TYPE APCst :
STRUCT
	Enable_b	:	BOOL	;	//	
	P1ZeroOffsetOutRangeAlm_b	:	BOOL	;	//	
	P1ZeroAdjOutRangeAlm_b	:	BOOL	;	//	
	P1SpanAdjOutRangeAlm_b	:	BOOL	;	//	
	P2ZeroOffsetOutRangeAlm_b	:	BOOL	;	//	
	P2ZeroAdjOutRangeAlm_b	:	BOOL	;	//	
	P2SpanAdjOutRangeAlm_b	:	BOOL	;	//	
	P1PressCtrlInterlockAlm_b	:	BOOL	;	//	
	P2PressCtrlInterlockAlm_b	:	BOOL	;	//	
	ValveOpenCtrlInterlockAlm_b	:	BOOL	;	//	
	ValveHoldCtrlInterlockAlm_b	:	BOOL	;	//	
	ValveCloseInterlockAlm_b	:	BOOL	;	//	
	AutoTeachingInterlockAlm_b	:	BOOL	;	//	
	P1DisconnectionAlm_b	:	BOOL	;	//	
	P2DisconnectionAlm_b	:	BOOL	;	//	
	PumpStopInterlockAlm_b	:	BOOL	;	//	
	AutoTeachingErr1Alm_b	:	BOOL	;	//	
	AutoTeachingErr2Alm_b	:	BOOL	;	//	
	Spare2_b	:	BOOL	;	//	
	Spare3_b	:	BOOL	;	//	
	Spare4_b	:	BOOL	;	//	
	Spare5_b	:	BOOL	;	//	
	Spare6_b	:	BOOL	;	//	
	Spare7_b	:	BOOL	;	//	
	Spare8_b	:	BOOL	;	//	
	Spare9_B	:	BOOL	;	//	
	SpareA_b	:	BOOL	;	//	
	SpareB_b	:	BOOL	;	//	
	SpareC_b	:	BOOL	;	//	
	SpareD_b	:	BOOL	;	//	
	SpareE_b	:	BOOL	;	//	
	SpareF_b	:	BOOL	;	//	
	PosMonOffsetSetting_Int	:	INT	;	//	-12000
	Spare3_Int	:	INT	;	//	
	Spare4_Int	:	INT	;	//	
	Spare5_Int	:	INT	;	//	
	Spare6_Int	:	INT	;	//	
	Spare7_Int	:	INT	;	//	
	Spare8_Int	:	INT	;	//	
	Spare9_Int	:	INT	;	//	
	SlowVccModeSetting_Usint	:	USINT	;	//	0,1
	ActiveControllerSetting_Usint	:	USINT	;	//	initial:0,0-255
	ControlModeSet_Usint	:	USINT	;	//	initial:0,0-255
	P1RangeUpLimitSet_Usint	:	USINT	;	//	initial:3,1-5
	P2RangeUpLimitSet_Usint	:	USINT	;	//	initial:5,1-5
	ControllerSelectFdbk_Usint	:	USINT	;	//	
	ControlModeFdbk_Usint	:	USINT	;	//	
	DisableInterlock_Usint	:	USINT	;	//	0,1
	HomingStatus_Usint	:	USINT	;	//	
	P1ZeroRst_Usint	:	USINT	;	//	0,1
	P1ZeroAdj_Usint	:	USINT	;	//	0,1
	P1SpanAdj_Usint	:	USINT	;	//	0,1
	P2ZeroRst_Usint	:	USINT	;	//	0,1
	P2ZeroAdj_Usint	:	USINT	;	//	0,1
	P2SpanAdj_Usint	:	USINT	;	//	0,1
	Spare16_Usint	:	USINT	;	//	
	Spare17_Usint	:	USINT	;	//	
	Spare18_Usint	:	USINT	;	//	
	Spare19_Usint	:	USINT	;	//	
	Spare20_Usint	:	USINT	;	//	
	SlowVccTargetPresSV_Real	:	REAL	;	//	0-93325.68
	ValveStatusThresholdSV_Real	:	REAL	;	//	initial:3.57,0.36-17.86
	Interlock1Setting_Real	:	REAL	;	//	initial:1.5,0-100
	Interlock2Setting_Real	:	REAL	;	//	initial:10,0.1-100
	Interlock3Setting_Real	:	REAL	;	//	initial:10,0.1-100
	IntegrationConstantIntlk3Set_Real	:	REAL	;	//	initial:100,0.1-100
	P1OffsetSetting_Real	:	REAL	;	//	initial:0,-15-15
	SlowVccRateSV_Real	:	REAL	;	//	initial:0.1,0.1-20
	SlowVccPIDSV_P_Real	:	REAL	;	//	initial:0.2,0.01-9.99
	SlowVccPIDSV_I_Real	:	REAL	;	//	initial:0.2,0.00-9.99
	SlowVccPIDSV_D_Real	:	REAL	;	//	initial:0.4,0.00-9.99
	SlowVccSensorPIDSV_D_Real	:	REAL	;	//	initial:1,0.00-9.99
	ProcessPointSV_Real	:	REAL	;	//	initial:0,0-93325.68
	PositionPointSV_Real	:	REAL	;	//	initial:0,0-100
	Controller1SV_P_Real	:	REAL	;	//	initial:2.0,0.01-9.99
	Controller1SV_I_Real	:	REAL	;	//	initial:0.5,0.00-9.99
	Controller1SV_D_Real	:	REAL	;	//	initial:0.3,0.00-9.99
	Controller1SensorSV_D_Real	:	REAL	;	//	initial:0.3,0.00-9.99
	Controller1CHSV_Real	:	REAL	;	//	initial:53.57,0.36-98.21
	Controller1CLSV_Real	:	REAL	;	//	initial:1.79,0.36-98.21
	Controller2SV_P_Real	:	REAL	;	//	initial:2.0,0.01-9.99
	Controller2SV_I_Real	:	REAL	;	//	initial:0.5,0.00-9.99
	Controller2SV_D_Real	:	REAL	;	//	initial:0.3,0.00-9.99
	Controller2SensorSV_D_Real	:	REAL	;	//	initial:0.3,0.00-9.99
	Controller2CHSV_Real	:	REAL	;	//	initial:53.57,0.36-98.21
	Controller2CLSV_Real	:	REAL	;	//	initial:1.79,0.36-98.21
	Controller3SV_P_Real_Copy	:	REAL	;	//	initial:2.0,0.01-9.99
	Controller3SV_I_Real_Copy	:	REAL	;	//	initial:0.5,0.00-9.99
	Controller3SV_D_Real_Copy	:	REAL	;	//	initial:0.3,0.00-9.99
	Controller3SensorSV_D_Real_Copy	:	REAL	;	//	initial:0.3,0.00-9.99
	Controller3CHSV_Real_Copy	:	REAL	;	//	initial:53.57,0.36-98.21
	Controller3CLSV_Real_Copy	:	REAL	;	//	initial:1.79,0.36-98.21
	Spare6_Real	:	REAL	;	//	
	Spare7_Real	:	REAL	;	//	
	Spare8_Real	:	REAL	;	//	
	Spare9_Real	:	REAL	;	//	
	Spare10_Real	:	REAL	;	//	
	P1PressurePV_Real	:	REAL	;	//	
	P2PressurePV_Real	:	REAL	;	//	
	PostionActualValueFdbk_Real	:	REAL	;	//	
	OffsetForController1_UDINT	:	UDINT	;	//	initial:0,-999-999
	OffsetForController2_UDINT	:	UDINT	;	//	
	OffsetForController3_UDINT	:	UDINT	;	//	
	P1SetAlarm_UDINT	:	UDINT	;	//	
	P2SetAlarm_UDINT	:	UDINT	;	//	
	InterlockAlarm_UDINT	:	UDINT	;	//	
	P1DisconnectionAlarm_UDINT	:	UDINT	;	//	
	P2DisconectionAlarm_UDINT	:	UDINT	;	//	
	ManufactureErr_UDINT	:	UDINT	;	//	
	Spare10_UDINT	:	UDINT	;	//	

END_STRUCT
END_TYPE
